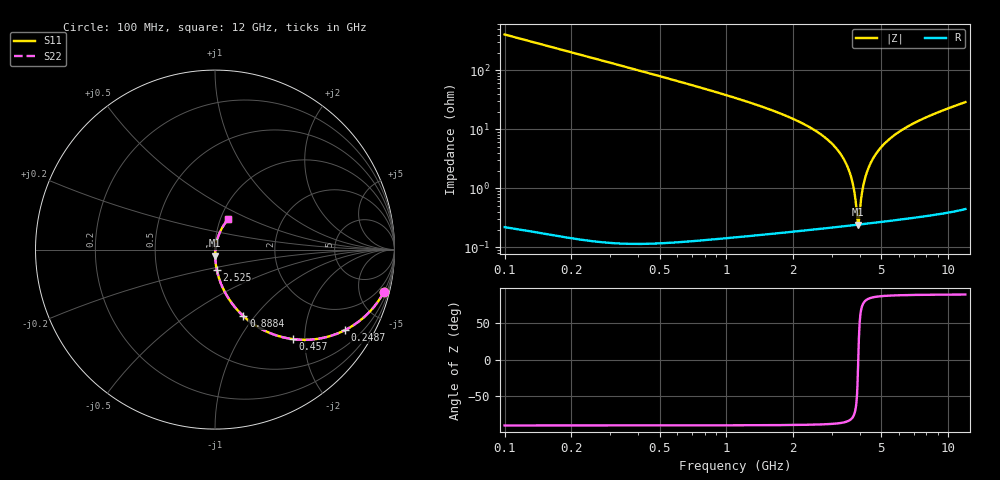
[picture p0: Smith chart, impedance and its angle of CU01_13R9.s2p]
! S-parameter model data by Modelithics Inc. support@modelithics.com 813-866-6335 Tampa FL USA
! S-Parameter data specifications:
! Substrate: 20-mil Rogers, substrate thickness, H=0.508mm, Dielectric constant, Er=3.75
! PCB Mounting Pad Footprint: Pad width, PadW=0.35mm , Pad length, PadL=0.30mm , Pad gap, PadG (edge-to-edge)=0.25mm , Reference planes=0.85mm apart
! Created Tue May  8 14:01:25 2018
# hz S ma R 50
! 2 Port Network Data from SP1.SP block
! freq  magS11  angS11  magS21  angS21  magS12  angS12  magS22  angS22
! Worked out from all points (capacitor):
!   801 points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, 100 MHz to 12 GHz, reference 50 ohm
!   read as one part in series: C = 3.93 pF near 159.5 MHz
!   lowest |Z| = 243 mohm at 3.938 GHz (marker M1)
!   series resonance near 3.942 GHz, so ESL is about 420 pH
!   S11 on the Smith chart (normalised r, x): 100 MHz: 0.99, -8.05; 248.8 MHz: 0.99, -3.23; 457 MHz: 0.99, -1.75; 888.4 MHz: 0.99, -0.88; 2.525 GHz: 0.99, -0.23; 12 GHz: 1.09, +0.39
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1e8  0.9707 -14.0  0.2396 76.0  0.2396 76.0  0.9707 -14.0
2.4875e8  0.8514 -31.8  0.5239 58.1  0.5239 58.1  0.8514 -31.8
4.57e8  0.6597 -49.1  0.7506 40.8  0.7506 40.8  0.6597 -49.1
6.50375e8  0.5214 -59.1  0.8522 30.8  0.8522 30.8  0.5214 -59.1
8.88375e8  0.4028 -66.9  0.914 22.9  0.914 22.9  0.4028 -66.9
2.09325e9  0.1548 -82.4  0.9861 6.9  0.9861 6.9  0.1548 -82.4
2.524625e9  0.1152 -84.8  0.9913 4.2  0.9913 4.2  0.1152 -84.8
3.3725e9  0.06064 -87.7  0.9959 0.2  0.9959 0.2  0.06064 -87.7
3.93775e9  0.0335 -87.8  0.997 -1.9  0.997 -1.9  0.0335 -87.8
4.071625e9  0.02777 -87.4  0.9971 -2.4  0.9971 -2.4  0.02777 -87.4
4.47325e9  0.01184 -81.4  0.9973 -3.7  0.9973 -3.7  0.01184 -81.4
4.741e9  0.003069 -37.1  0.9973 -4.5  0.9973 -4.5  0.003069 -37.1
4.785625e9  0.002596 -5.9  0.9973 -4.6  0.9973 -4.6  0.002596 -5.9
4.83025e9  0.003021 25.6  0.9973 -4.8  0.9973 -4.8  0.003021 25.6
5.023625e9  0.008651 66.8  0.9972 -5.3  0.9972 -5.3  0.008651 66.8
5.231875e9  0.01544 74.0  0.9971 -5.9  0.9971 -5.9  0.01544 74.0
5.574e9  0.02628 77.0  0.9968 -6.9  0.9968 -6.9  0.02628 77.0
6.05e9  0.0406 77.8  0.9962 -8.2  0.9962 -8.2  0.0406 77.8
6.883e9  0.06389 76.9  0.9948 -10.3  0.9948 -10.3  0.06389 76.9
8.04325e9  0.09378 74.8  0.9922 -13.2  0.9922 -13.2  0.09378 74.8
1.002162e10  0.141 70.7  0.9861 -17.8  0.9861 -17.8  0.141 70.7
1.2e10  0.1865 66.3  0.978 -22.3  0.978 -22.3  0.1865 66.3
